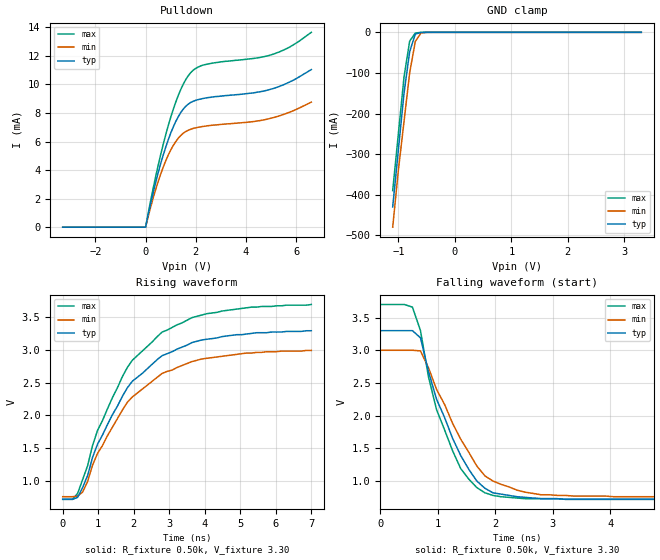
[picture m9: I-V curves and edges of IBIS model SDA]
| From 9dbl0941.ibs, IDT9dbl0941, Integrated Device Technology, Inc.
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|   Model SDA
[Model]   SDA
Model_type   I/O_open_drain
Polarity   Inverting
Enable   Active-High
Vinl =   0.80V
Vinh =   2.00V
Vmeas =   1.50V
Cref =   5.00pF
Rref =  0.000
Vref =   1.50V
C_comp   3.40pF   2.85pF   3.95pF
[Temperature Range]   27.00   70.00   0.000
[Voltage Range]   3.30V   3.00V   3.70V
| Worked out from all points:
|   slope of the pulldown table from 0 to 0.495 V, typ, clamps not added: 131 ohm
|   GND clamp passes 1 mA (typ) near -0.62 V on its own axis
|   rising waveform, R_fixture 0.50k, V_fixture 3.30: 20-80 % time 1.74ns typ, 1.76ns min, 1.73ns max; typ from 0.72 V to 3.29 V
|   falling waveform, R_fixture 0.50k, V_fixture 3.30: 20-80 % time 693ps typ, 785ps min, 596ps max; typ from 3.3 V to 0.72 V
[Pulldown]
| voltage   I(typ)   I(min)   I(max)
-3.3V     0A         0A         0A
0V        0A         0A         0A
500mV     3.8mA      3.19mA     4.32mA
900mV     6.11mA     5.04mA     7.1mA
1.2V      7.4mA      5.99mA     8.75mA
1.4V      8.03mA     6.42mA     9.64mA
1.8V      8.74mA     6.86mA     10.83mA
2.1V      8.94mA     7mA        11.22mA
2.5V      9.08mA     7.11mA     11.44mA
5.1V      9.72mA     7.68mA     12.13mA
5.7V      10.14mA    8.03mA     12.58mA
6.6V      11.04mA    8.76mA     13.65mA
[GND_clamp]
| voltage   I(typ)   I(min)   I(max)
  |-3.30   -3.78A   -3.64A   -3.87A
  |-3.20   -3.62A   -3.50A   -3.71A
  |-3.10   -3.47A   -3.35A   -3.55A
  |-3.00   -3.31A   -3.21A   -3.39A
  |-2.90   -3.16A   -3.06A   -3.23A
  |-2.80   -3.01A   -2.91A   -3.07A
  |-2.70   -2.85A   -2.77A   -2.91A
  |-2.60   -2.70A   -2.62A   -2.75A
  |-2.50   -2.54A   -2.48A   -2.59A
  |-2.40   -2.39A   -2.33A   -2.43A
  |-2.30   -2.24A   -2.19A   -2.27A
  |-2.20   -2.08A   -2.04A   -2.11A
  |-2.10   -1.93A   -1.90A   -1.95A
  |-2.00   -1.78A   -1.75A   -1.79A
  |-1.90   -1.62A   -1.61A   -1.63A
  |-1.80   -1.47A   -1.46A   -1.47A
  |-1.70   -1.32A   -1.32A   -1.32A
  |-1.60   -1.17A   -1.18A   -1.16A
  |-1.50   -1.02A   -1.03A   -1.00A
  |-1.40   -0.87A   -0.89A   -0.85A
  |-1.30   -0.72A   -0.75A   -0.69A
  |-1.20   -0.57A   -0.61A   -0.54A
-1.1V     -430mA     -480mA     -390mA
-1V       -290mA     -340mA     -250mA
-900mV    -150mA     -220mA     -110mA
-800mV    -47.73mA   -100mA     -21.74mA
-700mV    -4.4mA     -22.46mA   -1.7mA
-600mV    -390uA     -1.82mA    -190uA
-400mV    -1.59uA    -9.25uA    -420nA
3.3V      150pA      220pA      150pA
[Ramp]
| variable   typ   min   max
dV/dt_r   0.27/0.19n   0.21/0.19n   0.35/0.18n
dV/dt_f   0.27/0.21n   0.21/0.22n   0.35/0.20n
[Rising Waveform]
R_fixture = 0.50k
V_fixture = 3.30
V_fixture_min = 3.00
V_fixture_max = 3.70
| time   V(typ)   V(min)   V(max)
0s        720mV      760mV      720mV
280ps     720mV      760mV      720mV
420ps     750mV      770mV      810mV
560ps     900mV      830mV      1.02V
700ps     1.08V      990mV      1.23V
980ps     1.56V      1.42V      1.77V
1.82ns    2.42V      2.2V       2.73V
2.8ns     2.91V      2.64V      3.27V
4.06ns    3.16V      2.87V      3.55V
7ns       3.29V      2.99V      3.69V
[Falling Waveform]
R_fixture = 0.50k
V_fixture = 3.30
V_fixture_min = 3.00
V_fixture_max = 3.70
| time   V(typ)   V(min)   V(max)
0s        3.3V       3V         3.7V
560ps     3.3V       3V         3.66V
700ps     3.19V      2.99V      3.3V
840ps     2.67V      2.73V      2.59V
980ps     2.25V      2.4V       2.09V
1.4ns     1.39V      1.64V      1.19V
1.68ns    1V         1.23V      900mV
1.82ns    890mV      1.08V      820mV
2.8ns     730mV      790mV      730mV
7ns       720mV      760mV      720mV
